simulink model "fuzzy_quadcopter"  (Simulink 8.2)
settings: Solver=ode45  StartTime=0.0  StopTime=tsim  RelTol=1e-3
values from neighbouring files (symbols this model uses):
  I = 0.99    [Start.m]
  t2 = 200    [Start.m]
  t3 = 600    [Start.m]
  t4 = 1000    [Start.m]
  t5 = 1500    [Start.m]
  t6 = 2000    [Start.m]
  t7 = 2500    [Start.m]
  Td = 0.1    [Start.m]
  vx1 = -5    [Start.m]
  vx2 = -10    [Start.m]
  vx3 = -15    [Start.m]
  vx4 = 0    [Start.m]
  vx5 = 15    [Start.m]
  vx6 = 20    [Start.m]
  vx7 = 0    [Start.m]
  vy1 = 10    [Start.m]
  vy2 = -10    [Start.m]
  vy3 = 15    [Start.m]
  vy4 = 20    [Start.m]
  vy5 = 10    [Start.m]
  vy6 = -10    [Start.m]
  vy7 = 0    [Start.m]
libraries: fuzblock x2, simulink x1

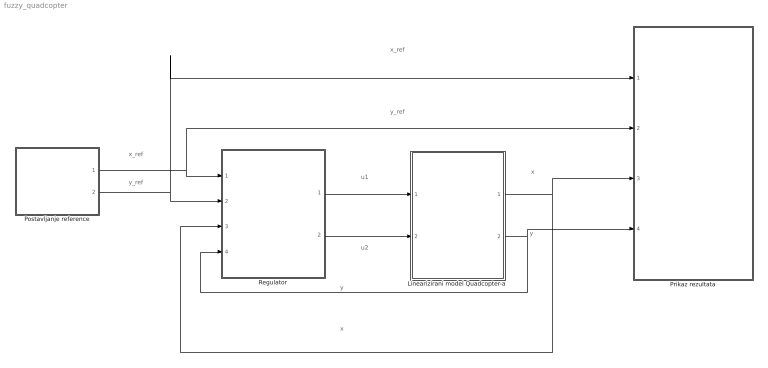
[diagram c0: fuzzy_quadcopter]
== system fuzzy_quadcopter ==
  note: x_ref
  note: y_ref
  note: y
  note: x
  note: u1
  note: u2
  note: x
  note: y
  note: x_ref
  note: y_ref
  "Linearizirani model Quadcopter-a " : Subsystem
  Postavljanje reference : Subsystem
  Prikaz rezultata : Subsystem
  Regulator : Subsystem
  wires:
  Postavljanje reference/2(y_ref) -> Prikaz rezultata/1(y_ref), Regulator/2(y_ref)
  Postavljanje reference/1(x_ref) -> Regulator/1(x_ref), Prikaz rezultata/2(x_ref)
  "Linearizirani model Quadcopter-a "/2(y) -> Regulator/4(y), Prikaz rezultata/4(y)
  "Linearizirani model Quadcopter-a "/1(x) -> Regulator/3(x), Prikaz rezultata/3(x)
  Regulator/1(u1) -> "Linearizirani model Quadcopter-a "/1(u1)
  Regulator/2(u2) -> "Linearizirani model Quadcopter-a "/2(u2)

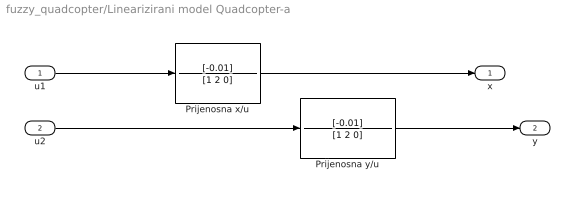
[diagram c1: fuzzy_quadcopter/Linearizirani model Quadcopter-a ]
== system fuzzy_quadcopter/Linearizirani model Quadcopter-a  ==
  u1 : Inport
  u2 : Inport  Port=2
  Prijenosna x/u : TransferFcn  Numerator=[-0.01]  Denominator=[1 2 0]
  Prijenosna y/u : TransferFcn  Numerator=[-0.01]  Denominator=[1 2 0]
  x : Outport
  y : Outport  Port=2
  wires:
  Prijenosna x/u/1 -> x/1
  u2/1 -> Prijenosna y/u/1
  u1/1 -> Prijenosna x/u/1
  Prijenosna y/u/1 -> y/1

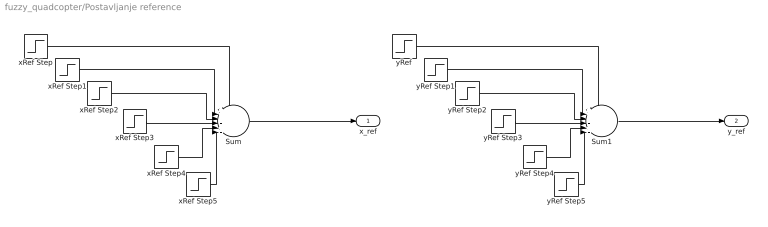
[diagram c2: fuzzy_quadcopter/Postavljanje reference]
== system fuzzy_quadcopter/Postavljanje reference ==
  Sum : Sum  Inputs=++++++|  RndMeth=Nearest
  Sum1 : Sum  Inputs=++++++|  RndMeth=Nearest
  xRef Step : Step  Time=t2  Before=vx1  After=vx2  SampleTime=0
  xRef Step1 : Step  Time=t3  After=vx3-vx2  SampleTime=0
  xRef Step2 : Step  Time=t4  After=vx4-vx3  SampleTime=0
  xRef Step3 : Step  Time=t5  After=vx5-vx4  SampleTime=0
  xRef Step4 : Step  Time=t6  After=vx6-vx5  SampleTime=0
  xRef Step5 : Step  Time=t7  After=vx7-vx6  SampleTime=0
  yRef : Step  Time=t2  Before=vy1  After=vy2  SampleTime=0
  yRef Step1 : Step  Time=t3  After=vy3-vy2  SampleTime=0
  yRef Step2 : Step  Time=t4  After=vy4-vy3  SampleTime=0
  yRef Step3 : Step  Time=t5  After=vy5-vy4  SampleTime=0
  yRef Step4 : Step  Time=t6  After=vy6-vy5  SampleTime=0
  yRef Step5 : Step  Time=t7  After=vy7-vy6  SampleTime=0
  x_ref : Outport
  y_ref : Outport  Port=2
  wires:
  Sum1/1 -> y_ref/1
  xRef Step/1 -> Sum/1
  yRef Step1/1 -> Sum1/2
  yRef Step2/1 -> Sum1/3
  xRef Step2/1 -> Sum/3
  xRef Step5/1 -> Sum/6
  yRef Step3/1 -> Sum1/4
  yRef Step4/1 -> Sum1/5
  xRef Step1/1 -> Sum/2
  yRef Step5/1 -> Sum1/6
  Sum/1 -> x_ref/1
  xRef Step4/1 -> Sum/5
  xRef Step3/1 -> Sum/4
  yRef/1 -> Sum1/1

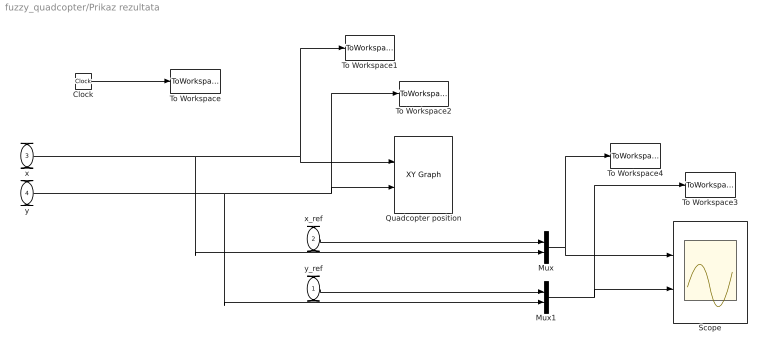
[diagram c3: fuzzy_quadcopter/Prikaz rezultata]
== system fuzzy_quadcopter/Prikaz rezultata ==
  y_ref : Inport
  x_ref : Inport  Port=2
  x : Inport  Port=3
  y : Inport  Port=4
  Clock : Clock
  Mux : Mux  Inputs=2
  Mux1 : Mux  Inputs=2
  Quadcopter position : simulink/Sinks/XY Graph  xmin=-32  xmax=32  ymin=-32  ymax=32  st=-1
  Scope : Scope  NumInputPorts=2
  To Workspace : ToWorkspace  VariableName=t  SampleTime=-1
  To Workspace1 : ToWorkspace  VariableName=x  SampleTime=-1
  To Workspace2 : ToWorkspace  VariableName=y  SampleTime=-1
  To Workspace3 : ToWorkspace  VariableName=y_1  SampleTime=-1
  To Workspace4 : ToWorkspace  VariableName=x_1  SampleTime=-1
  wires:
  y/1 -> Mux1/2, Quadcopter position/2, To Workspace2/1
  y_ref/1 -> Mux1/1
  x_ref/1 -> Mux/1
  x/1 -> Quadcopter position/1, To Workspace1/1, Mux/2
  Mux1/1 -> Scope/2, To Workspace3/1
  Clock/1 -> To Workspace/1
  Mux/1 -> Scope/1, To Workspace4/1

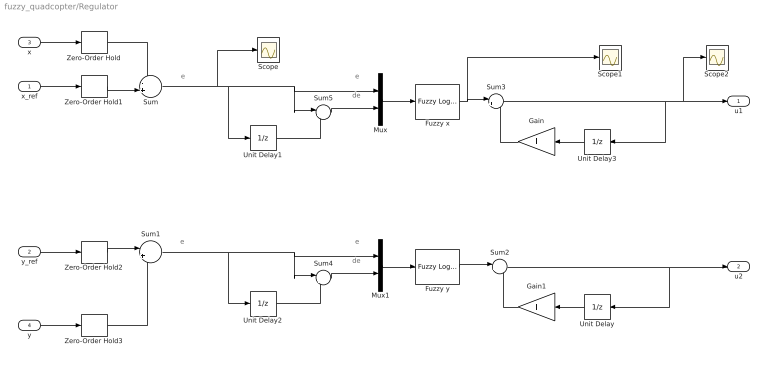
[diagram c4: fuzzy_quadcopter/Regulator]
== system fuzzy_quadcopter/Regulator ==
  note: e
  note: de
  note: e
  note: de
  note: e
  note: e
  x_ref : Inport
  y_ref : Inport  Port=2
  x : Inport  Port=3
  y : Inport  Port=4
  Fuzzy x : fuzblock/Fuzzy Logic  Controller  fis=fuzzy_projekt
  Fuzzy y : fuzblock/Fuzzy Logic  Controller  fis=fuzzy_projekt
  Gain : Gain  Gain=I
  Gain1 : Gain  Gain=I
  Mux : Mux  Inputs=2
  Mux1 : Mux  Inputs=2
  Scope : Scope
  Scope1 : Scope
  Scope2 : Scope
  Sum : Sum  Inputs=-+|  RndMeth=Nearest
  Sum1 : Sum  Inputs=|+-  RndMeth=Nearest
  Sum2 : Sum  Inputs=|++
  Sum3 : Sum  Inputs=|++
  Sum4 : Sum  Inputs=|+-
  Sum5 : Sum  Inputs=|+-
  Unit Delay : UnitDelay  SampleTime=Td
  Unit Delay1 : UnitDelay  SampleTime=-1
  Unit Delay2 : UnitDelay  SampleTime=-1
  Unit Delay3 : UnitDelay  SampleTime=Td
  Zero-Order Hold{,1..3} (4 alike) : ZeroOrderHold  SampleTime=Td
  u1 : Outport
  u2 : Outport  Port=2
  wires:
  Sum/1 -> Unit Delay1/1, Sum5/1, Mux/1, Scope/1
  x/1 -> Zero-Order Hold/1
  x_ref/1 -> Zero-Order Hold1/1
  y_ref/1 -> Zero-Order Hold2/1
  y/1 -> Zero-Order Hold3/1
  Mux/1 -> Fuzzy x/1
  Fuzzy y/1 -> Sum2/1
  Sum5/1 -> Mux/2
  Unit Delay1/1 -> Sum5/2
  Zero-Order Hold/1 -> Sum/1
  Zero-Order Hold1/1 -> Sum/2
  Zero-Order Hold2/1 -> Sum1/1
  Zero-Order Hold3/1 -> Sum1/2
  Unit Delay/1 -> Gain1/1
  Sum2/1 -> Unit Delay/1, u2/1
  Unit Delay3/1 -> Gain/1
  Sum3/1 -> Unit Delay3/1, Scope2/1, u1/1
  Fuzzy x/1 -> Scope1/1, Sum3/1
  Gain/1 -> Sum3/2
  Gain1/1 -> Sum2/2
  Sum1/1 -> Unit Delay2/1, Sum4/1, Mux1/1
  Mux1/1 -> Fuzzy y/1
  Sum4/1 -> Mux1/2
  Unit Delay2/1 -> Sum4/2
